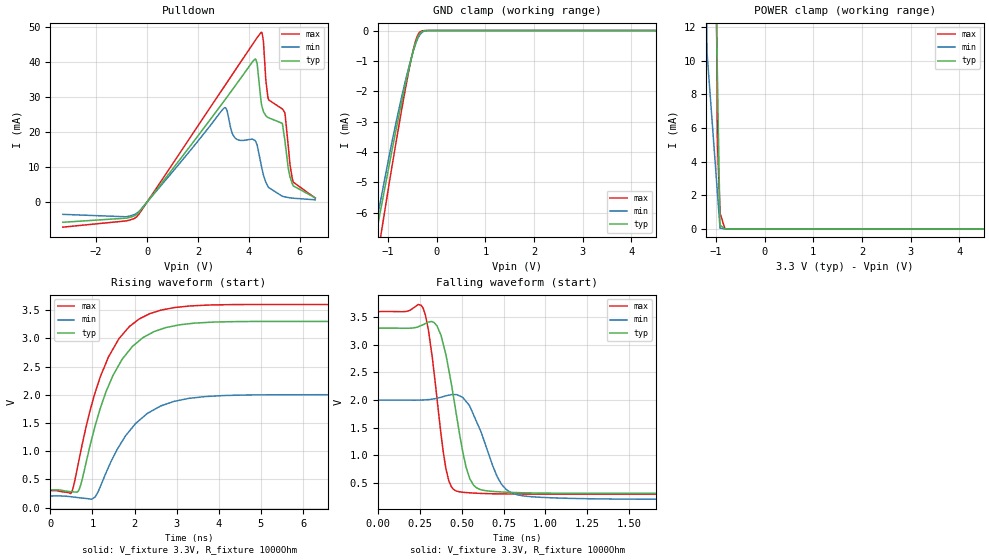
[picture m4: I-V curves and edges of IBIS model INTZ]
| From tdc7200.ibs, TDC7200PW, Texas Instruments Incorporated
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|   Model  INTZ
[Model]   INTZ
Model_type   I/O_open_drain
Polarity   Non-Inverting
Enable   Active-Low
Vinl = .8
Vinh = 2
Vmeas = 1.65
Vref = 3.3
Cref = 15pF
Rref = 1000
|   typ   min   max
|   (nom PVT)   (fast PVT)   (slow PVT)
C_comp   0.157p   0.149p   0.168p
|C_comp (ON/Low state)   0.157p   0.149p   0.168p
|C_comp (OFF state)   0.215p   0.213p   0.226p
[Voltage Range]   3.3   2   3.6
[Temperature Range]   27   125   -40
[Pullup Reference]   3.3   2   3.6
[Pulldown Reference]   0   0   0
[Power Clamp Reference]   3.3   2   3.6
[GND Clamp Reference]   0   0   0
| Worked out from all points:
|   slope of the pulldown table from 0 to 0.495 V, typ, clamps not added: 106 ohm
|   GND clamp passes 1 mA (typ) near -0.53 V on its own axis
|   POWER clamp passes 1 mA (typ) near -0.92 V on its own axis
|   falling waveform, V_fixture 3.3V, R_fixture 1000Ohm: 20-80 % time 104ps typ, 138ps min, 78.9ps max; typ from 3.3 V to 0.314 V
|   rising waveform, V_fixture 3.3V, R_fixture 1000Ohm: 20-80 % time 899ps typ, 965ps min, 875ps max; typ from 0.314 V to 3.3 V
[Pulldown]
|   Voltage   I(typ)   I(min)   I(max)
-3.3V     -5.754mA   -3.494mA   -7.142mA
-399.3mV  -3.494mA   -3.139mA   -4.139mA
3.046V    29.06mA    26.92mA    33.14mA
3.442V    33mA       18.38mA    37.43mA
4.244V    40.79mA    17.49mA    46.09mA
4.481V    28.29mA    10.47mA    48.41mA
4.561V    25.93mA    7.852mA    46.14mA
4.769V    24.04mA    4.166mA    29.15mA
5.303V    22.47mA    1.679mA    26.58mA
5.412V    17.21mA    1.488mA    25.24mA
5.739V    4.61mA     1.105mA    5.67mA
6.6V      1.213mA    653.2uA    1.146mA
[GND Clamp]
|   Voltage   I(typ)   I(min)   I(max)
-3.3V     -26.21mA   -27.51mA   -28.97mA
-1.419V   -8.231mA   -7.972mA   -9.48mA
-1.181V   -6.174mA   -5.854mA   -7.104mA
-973.5mV  -4.425mA   -4.115mA   -5.024mA
-716.1mV  -2.339mA   -2.167mA   -2.587mA
-518.1mV  -911uA     -887.1uA   -908.9uA
-448.8mV  -500.4uA   -522.5uA   -439.7uA
-399.3mV  -267.5uA   -310.6uA   -195.1uA
-359.7mV  -134.4uA   -180.9uA   -77.93uA
-310.2mV  -42.62uA   -76.19uA   -17.32uA
-112.2mV  -37.07nA   -516.5nA   0A
6.6V      0A         0A         0A
[POWER Clamp]
|   Voltage   I(typ)   I(min)   I(max)
-3.3V     1.595A     1.341A     1.768A
-1.419V   146.1mA    82.72mA    196.7mA
-1.181V   44.19mA    10.5mA     95.83mA
-967.9mV  9.076mA    2.153mA    5.162mA
-914.1mV  226.3uA    49.04uA    939.9uA
-815.1mV  13.13uA    5.709uA    25.28uA
-765.6mV  3.144uA    1.954uA    4.018uA
6.6V      0A         0A         0A
[Ramp]
R_load = 1000
|   typ   min   max
dV/dt_r   1.79139/8.98607e-10   1.07616/9.65418e-10   1.97946/8.74785e-10
dV/dt_f   1.79135/1.04254e-10   1.07614/1.37507e-10   1.97942/7.88798e-11
[Falling Waveform]
V_fixture = 3.3V
V_fixture_min = 2V
V_fixture_max = 3.6V
R_fixture = 1000Ohm
C_fixture = 0F
|   Time   V(typ)   V(min)   V(max)
0s        3.3V       2V         3.6V
256.7ps   3.346V     2V         3.715V
300ps     3.411V     2.008V     3.277V
352.9ps   3.337V     2.032V     2.002V
422.7ps   2.541V     2.088V     539mV
507.3ps   1.043V     2.043V     334.3mV
560.1ps   516.4mV    1.806V     321.3mV
767.6ps   334.9mV    379.8mV    303.3mV
1.129ns   315.6mV    225mV      300.8mV
19.9ns    314.4mV    206.4mV    301mV
[Rising Waveform]
V_fixture = 3.3V
V_fixture_min = 2V
V_fixture_max = 3.6V
R_fixture = 1000Ohm
C_fixture = 0F
|   Time   V(typ)   V(min)   V(max)
0s        314.4mV    206.4mV    300.9mV
483.3ps   283.3mV    194.1mV    250.1mV
659.5ps   287mV      177.5mV    763.8mV
1.065ns   1.45V      188.1mV    2.038V
1.381ns   2.155V     714.7mV    2.671V
1.704ns   2.629V     1.174V     3.06V
1.955ns   2.862V     1.428V     3.255V
2.629ns   3.163V     1.804V     3.502V
4.721ns   3.299V     1.998V     3.6V
19.9ns    3.3V       2V         3.6V
